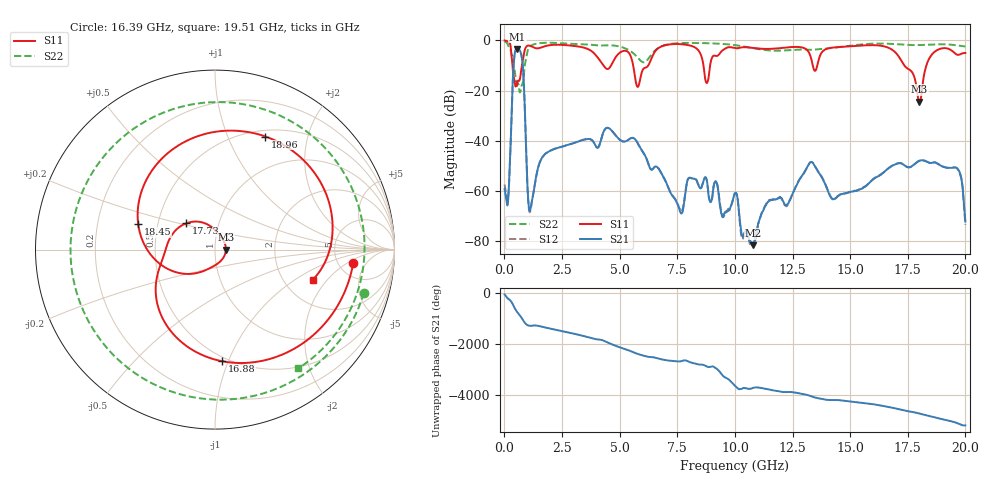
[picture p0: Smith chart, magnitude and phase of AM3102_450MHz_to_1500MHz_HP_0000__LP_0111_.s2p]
!Agilent Technologies,E8364B,MY43040894,A.07.50.67
!Agilent E8364B: A.07.50.67
!Date: Thursday, January 11, 2018 05:16:24
!Correction: S11(Full 2 Port(1,2))
!S21(Full 2 Port(1,2))
!S12(Full 2 Port(1,2))
!S22(Full 2 Port(1,2))
!S2P File: Measurements: S11, S21, S12, S22:
# Hz S  dB  R 50
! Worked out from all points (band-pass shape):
!   1601 points, 10 MHz to 20 GHz, reference 50 ohm
!   highest |S21| = -3.38 dB at 559.7 MHz (marker M1); lowest = -81.5 dB at 10.79 GHz (marker M2)
!   |S21| within 3 dB of the highest: 434.1 MHz to 749 MHz (314.9 MHz wide, 53.2 % of centre)
!   lowest |S11| = -24.3 dB at 18 GHz (marker M3), VSWR 1.13, Z = 56.5 + j0.0558 ohm
!   |S11| at or under -10 dB: 349.4 MHz to 763 MHz (413.6 MHz wide, 74.4 % of centre); 5.587 GHz to 6.239 GHz (651.9 MHz wide, 11 % of centre); 17.35 GHz to 18.31 GHz (953.2 MHz wide, 5.35 % of centre)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
!   |S22| runs from -20.7 to -0.4 dB; largest |S21 - S12| = 0.0015
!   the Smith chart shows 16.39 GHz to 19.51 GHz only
!   S11 on the Smith chart (normalised r, x): 16.39 GHz: 6.90, -2.53; 16.88 GHz: 0.47, -0.95; 17.73 GHz: 0.70, +0.21; 18.45 GHz: 0.39, +0.14; 18.96 GHz: 0.57, +1.38; 19.51 GHz: 2.85, -1.43
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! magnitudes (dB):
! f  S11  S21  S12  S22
! 10 MHz  0.0  -59.1  -57.4  -0.4
! 172.4 MHz  -0.6  -62.6  -61.2  -2.2
! 559.7 MHz  -17.1  -3.4  -3.4  -17.2
! 784.6 MHz  -8.9  -8.7  -8.7  -17.3
! 1.109 GHz  -2.2  -67.8  -68.2  -2.4
! 3.346 GHz  -2.7  -39.8  -39.8  -1.6
! 5.782 GHz  -18.5  -40.9  -40.9  -6.9
! 6.682 GHz  -3.1  -50.9  -50.9  -3.0
! 7.656 GHz  -1.5  -68.7  -68.2  -1.1
! 8.781 GHz  -17.0  -55.6  -55.8  -1.1
! 10.01 GHz  -3.1  -60.7  -60.9  -1.9
! 10.79 GHz  -3.0  -81.5  -81.8  -3.1
! 13.34 GHz  -8.4  -48.4  -48.4  -3.8
! 16.39 GHz  -2.2  -53.0  -53.0  -1.3
! 16.68 GHz  -3.0  -50.8  -50.8  -1.4
! 16.88 GHz  -4.1  -49.6  -49.7  -1.5
! 17.73 GHz  -13.3  -49.8  -49.8  -1.9
! 18 GHz  -24.3  -47.9  -47.9  -1.9
! 18.45 GHz  -6.9  -48.8  -48.7  -1.7
! 18.96 GHz  -3.2  -50.0  -50.0  -1.6
! 19.51 GHz  -4.9  -50.5  -50.6  -1.9
! 20 GHz  -5.0  -72.1  -73.4  -2.4
